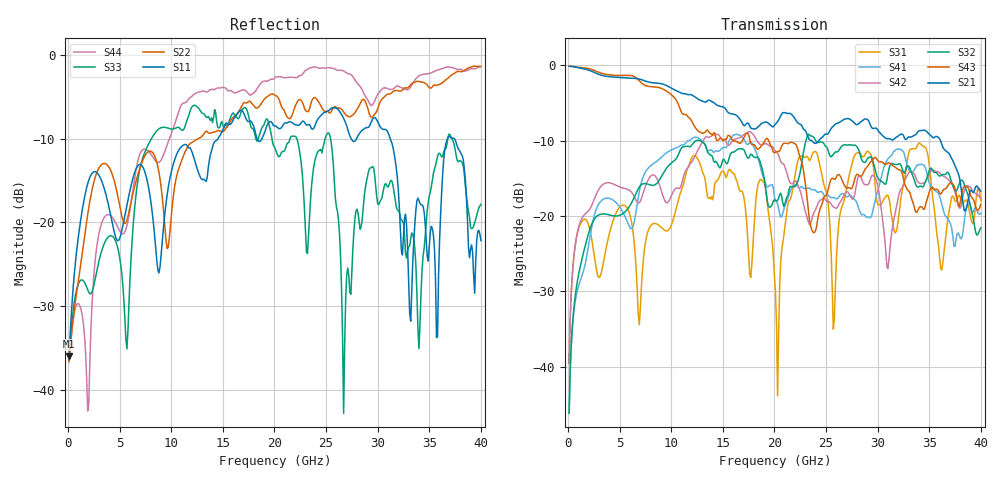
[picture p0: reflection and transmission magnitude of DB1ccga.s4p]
! ADC12DJ3200QML-SP
! 196-pin NWE package
! CCGA Ceramic Package with columns (ceramic column grid array)
! Texas Instruments 4/21/2021
! Single-ended  S-parameters
! PORT#  PORT_NAME  NET_NAME
! PORT1:  DAxN.DIEBUMP DAxN
! PORT2:  DAxN.BGA  DAxN
! PORT3:  DAxP.DIEBUMP DAxP
! PORT4:  DAxP.BGA  DAxP
! Touchstone Ver. 1.0
! Number of ports is 4
# Hz	S	MA	R	50.000000
! SCATTERING PARAMETERS  :
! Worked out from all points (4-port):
!   400 points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, 100 MHz to 40 GHz, reference 50 ohm
!   strongest paths, dB at 100 MHz, 10.1 GHz, 20.1 GHz, 30.1 GHz, 40 GHz:
!     S21: -0.1, -3.1, -7.8, -8.8, -16.7
!     S43: -0.1, -4.0, -11.5, -12.8, -18.5
!     S32: -46.2, -12.9, -18.0, -15.1, -21.6
!     S42: -39.5, -17.0, -11.4, -16.7, -17.7
!     S41: -46.2, -11.2, -17.8, -16.2, -19.6
!     S31: -39.5, -20.9, -30.3, -18.6, -18.0
!   lowest |S11| = -36.0 dB at 100 MHz (marker M1), VSWR 1.03, Z = 51.5 + j0.574 ohm
!   |S11| at or under -10 dB: start of sweep to 14.53 GHz; 31.21 GHz to 36.77 GHz (5.561 GHz wide, 16.4 % of centre); 37.42 GHz to end of sweep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
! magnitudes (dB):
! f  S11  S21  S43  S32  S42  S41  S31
! 100 MHz  -36.0  -0.1  -0.1  -46.2  -39.5  -46.2  -39.5
! 12.4 GHz  -13.2  -4.3  -8.4  -10.0  -11.8  -9.5  -12.1
! 20.3 GHz  -8.7  -7.5  -11.5  -17.9  -11.7  -18.4  -43.9
! 25.3 GHz  -6.6  -8.9  -15.9  -11.8  -18.1  -17.4  -19.8
! 26.7 GHz  -7.6  -7.2  -15.7  -10.6  -17.3  -17.1  -18.1
! 29.2 GHz  -8.5  -7.6  -13.0  -12.2  -15.5  -20.2  -11.6
! 40 GHz  -22.2  -16.7  -18.5  -21.6  -17.7  -19.6  -18.0
